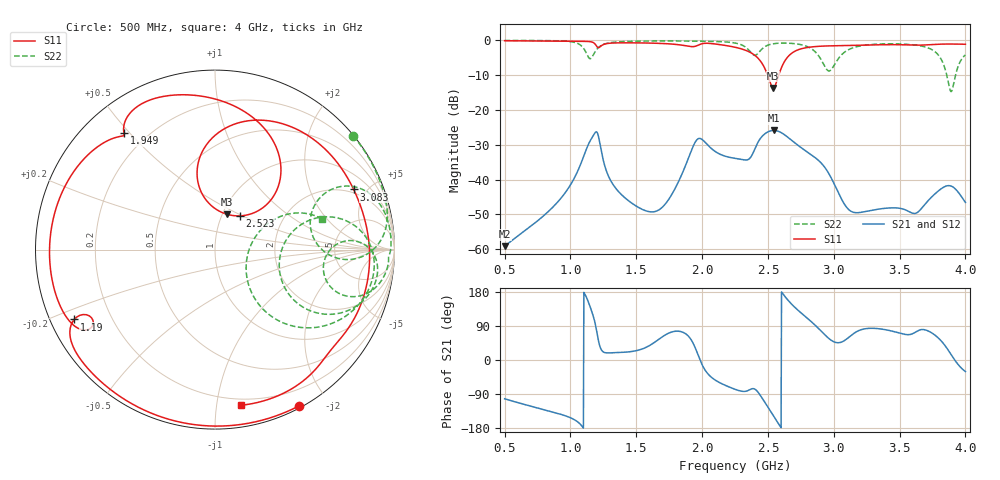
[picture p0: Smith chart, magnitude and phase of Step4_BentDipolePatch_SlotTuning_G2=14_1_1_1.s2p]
! TOUCHSTONE file generated by CST MICROWAVE STUDIO
! Date and time: Wed May 20 12:59:06 2020
! Project name: DualBand_DualMode_Antenna_FD_SteppedDesign.cst
! Parameters = {FPL=20; FPW=20; L=50; ST=10; SW=30; W=52; WF=7; ext=10; gap=1; inset=13}
! Header version: 2015
! Port assignment regex: !\s*Touchstone port\s*([0-9]+)\s*=\s*CST MWS port\s*([0-9]+)\s*\(\"(.*)\"\)(\s*mode\s*([0-9]+))?.*
! Touchstone port assignment:
! Touchstone port 1 = CST MWS port 1 ("")
! Touchstone port 2 = CST MWS port 2 ("")
# GHz S MA R 50
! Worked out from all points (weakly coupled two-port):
!   1006 points, 500 MHz to 4 GHz, reference 50 ohm
!   highest |S21| = -25.87 dB at 2.544 GHz (marker M1); lowest = -59.1 dB at 500 MHz (marker M2)
!   lowest |S11| = -13.7 dB at 2.541 GHz (marker M3), VSWR 1.52, Z = 52.3 + j21.6 ohm
!   |S11| at or under -10 dB: 2.498 GHz to 2.582 GHz (84.06 MHz wide, 3.31 % of centre)
!   |S22| runs from -14.7 to 0.0 dB; largest |S21 - S12| = 3.4e-05
!   S11 on the Smith chart (normalised r, x): 500 MHz: 0.02, -1.67; 1.19 GHz: 0.07, -0.23; 1.949 GHz: 0.12, +0.48; 2.523 GHz: 1.21, +0.48; 3.083 GHz: 1.78, +4.09; 4 GHz: 0.15, -1.17
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0.5  0.9886 -61.8  0.001107 -102.3  0.001107 -102.3  0.9965 39.4
0.899  0.9781 -111.1  0.004676 -140.5  0.004676 -140.5  0.987 14.3
1.0845  0.9706 -135.0  0.01798 -173.2  0.01798 -173.2  0.831 -2.4
1.1475  0.9601 -144.8  0.03542 142.6  0.03541 142.6  0.5467 9.7
1.1895  0.8754 -153.6  0.04776 93.7  0.04776 93.7  0.6969 27.2
1.3505  0.9205 -162.8  0.007261 19.5  0.007258 19.5  0.9484 16.1
1.669  0.9073 157.2  0.003647 54.1  0.003648 54.1  0.9816 5.4
1.949  0.8231 128.0  0.03485 31.2  0.03485 31.2  0.9703 -1.9
2.25  0.7974 80.3  0.02022 -77.3  0.02022 -77.3  0.917 -13.5
2.397  0.6173 54.1  0.02656 -76.3  0.02656 -76.3  0.6116 -9.2
2.523  0.2323 53.9  0.05029 -137.0  0.05029 -137.0  0.8803 -1.2
2.5405  0.2077 72.0  0.05086 -146.7  0.05086 -146.7  0.8938 -2.7
2.544  0.2085 76.1  0.05089 -148.7  0.05089 -148.7  0.8959 -3.0
2.635  0.5292 98.8  0.04287 165.1  0.04287 165.1  0.9142 -10.1
2.8345  0.8068 57.5  0.0224 99.6  0.0224 99.6  0.7496 -28.7
2.957  0.8332 39.4  0.01273 58.5  0.01273 58.5  0.367 -12.7
3.083  0.8421 23.4  0.004381 51.7  0.004382 51.7  0.6792 15.5
3.419  0.8682 -15.6  0.003914 78.1  0.003913 78.1  0.8933 -7.5
3.622  0.8544 -38.0  0.003285 73.8  0.003289 73.8  0.856 -21.2
3.776  0.8782 -53.9  0.006421 63.6  0.006421 63.6  0.6703 -40.6
3.8915  0.8866 -67.7  0.008085 14.4  0.008085 14.4  0.1838 -11.9
4  0.8794 -80.5  0.004703 -30.4  0.004703 -30.4  0.6183 16.2
